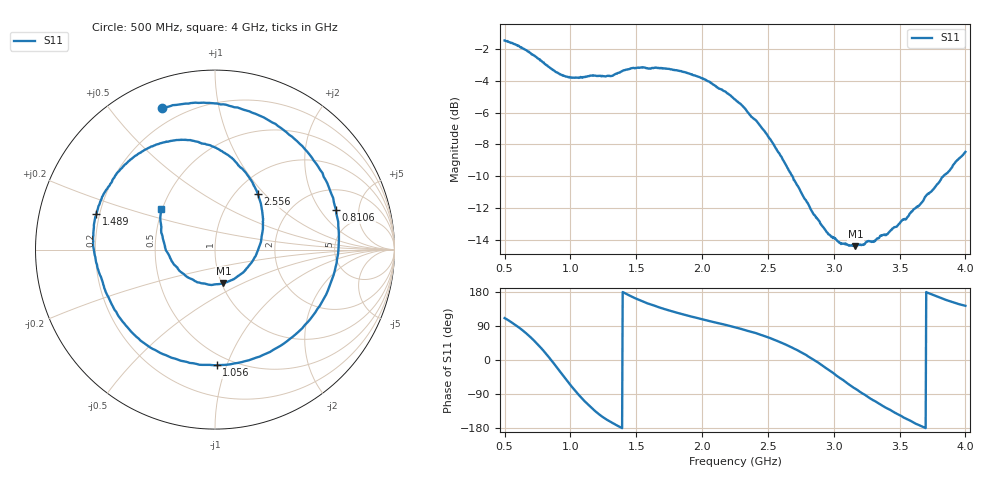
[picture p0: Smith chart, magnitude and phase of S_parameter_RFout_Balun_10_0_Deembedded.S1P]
!Agilent Technologies,E5071B,MY42403504,A.06.51
!Date: Wed Feb 26 14:57:15 2014
!Data & Calibration Information:
!Freq	S11:SOLT1(ON)
# Hz S dB R 50
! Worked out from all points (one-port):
!   801 points, 500 MHz to 4 GHz, reference 50 ohm
!   lowest |S11| = -14.4 dB at 3.164 GHz (marker M1), VSWR 1.47, Z = 51.1 - j19.7 ohm
!   |S11| at or under -10 dB: 2.687 GHz to 3.831 GHz (1.144 GHz wide, 35.1 % of centre)
!   S11 on the Smith chart (normalised r, x): 500 MHz: 0.13, +0.69; 810.6 MHz: 3.20, +2.85; 1.056 GHz: 0.42, -0.92; 1.489 GHz: 0.19, +0.14; 2.556 GHz: 1.26, +0.91; 4 GHz: 0.49, +0.26
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5e8  -1.49 110.6
5.91875e8  -1.79 89.9
6.6625e8  -2.11 69.7
7.3625e8  -2.51 46.8
8.10625e8  -2.98 18.2
8.71875e8  -3.36 -8.2
9.375e8  -3.67 -38.0
9.9875e8  -3.81 -65.4
1.055625e9  -3.82 -89.2
1.12125e9  -3.76 -113.3
1.2e9  -3.72 -138.3
1.274375e9  -3.72 -157.0
1.375e9  -3.50 -176.6
1.48875e9  -3.23 163.4
1.655e9  -3.20 141.2
1.8125e9  -3.37 124.5
2.018125e9  -3.93 106.0
2.25e9  -5.18 86.2
2.41625e9  -6.56 70.1
2.55625e9  -8.20 52.3
2.6875e9  -10.01 32.1
2.88875e9  -12.78 -8.7
3.125e9  -14.32 -66.7
3.164375e9  -14.36 -75.8
3.348125e9  -13.79 -116.0
3.5625e9  -12.52 -156.9
3.715625e9  -11.08 176.8
4e9  -8.46 143.0
